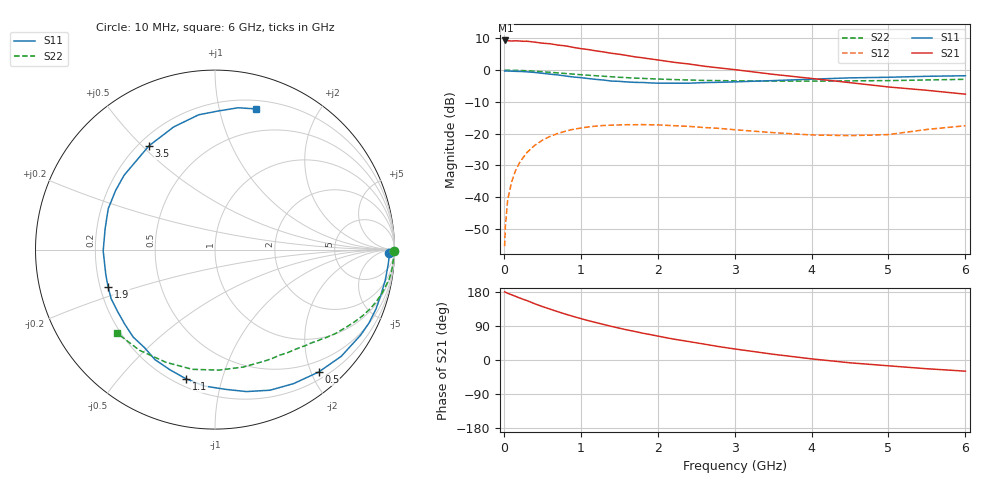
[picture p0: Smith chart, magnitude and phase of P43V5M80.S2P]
! SIEMENS Small Signal Semiconductors
! BFP182
! Si NPN RF Bipolar Junction Transistor in SOT143
! VCE = 3.5 V  IC = 0.8 mA
! Common Emitter S-Parameters:  March  1996
# GHz  S  MA  R  50
!  f  S11  S21  S12  S22
! GHz  MAG  ANG  MAG  ANG  MAG  ANG  MAG  ANG
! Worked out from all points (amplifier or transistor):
!   36 points, 10 MHz to 6 GHz, reference 50 ohm
!   highest |S21| = 9.3 dB at 20 MHz (marker M1)
!   |S21| within 3 dB of that: start of sweep to 1.13 GHz
!   unconditionally stable (mu >= 1): 2.769 GHz to end of sweep
!   at 250 MHz: K = 0.09, MSG = 18.3 dB, |S12| = -27.5 dB
!   at 1.4 GHz: K = 0.52, MSG = 11.3 dB, |S12| = -17.3 dB
!   at 6 GHz: K = 1.11, MAG = 2.9 dB, |S12| = -17.5 dB
!   S11 on the Smith chart (normalised r, x): 10 MHz: 49, -27; 500 MHz: 0.31, -2.12; 1.1 GHz: 0.24, -0.77; 1.9 GHz: 0.23, -0.16; 3.5 GHz: 0.24, +0.52; 6 GHz: 0.28, +1.30
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0.01  0.9692 -1.0  2.885 179.6  0.0017 85.5  0.9986 -0.3
0.02  0.9717 -2.0  2.934 179.1  0.0035 83.0  0.9999 -0.8
0.05  0.9682 -5.1  2.911 176.1  0.0091 89.3  0.9983 -1.8
0.1  0.964 -10.0  2.874 172.2  0.0172 83.3  0.9943 -3.7
0.15  0.9584 -15.5  2.897 168.2  0.0259 79.9  0.9931 -5.6
0.3  0.941 -30.4  2.852 156.8  0.0505 71.1  0.9777 -11.0
0.4  0.921 -40.2  2.762 148.5  0.0654 64.7  0.9626 -14.5
0.5  0.8937 -49.8  2.66 141.1  0.0788 58.5  0.9447 -17.8
0.6  0.8656 -59.6  2.604 134.3  0.0907 53.0  0.9263 -20.7
0.8  0.8102 -77.5  2.413 121.1  0.1094 43.1  0.8855 -26.1
1.1  0.7378 -102.6  2.107 103.7  0.128 30.4  0.8319 -32.8
1.3  0.6985 -118.6  1.931 93.6  0.1349 23.1  0.8018 -36.8
1.5  0.6672 -133.1  1.781 84.0  0.1374 17.1  0.7725 -40.4
1.9  0.6307 -160.9  1.505 67.2  0.1383 7.0  0.7338 -47.0
2.2  0.623 -179.4  1.335 55.4  0.1339 1.4  0.7113 -51.8
2.8  0.6441 149.4  1.085 35.2  0.1214 -6.1  0.6852 -62.2
3.5  0.6852 122.5  0.86 15.2  0.104 -7.4  0.6731 -76.5
4  0.7212 108.6  0.741 3.0  0.0956 -2.9  0.6717 -88.2
4.5  0.7566 96.9  0.636 -7.4  0.0933 3.0  0.6789 -100.7
5  0.7732 88.4  0.544 -15.3  0.0969 13.1  0.6848 -113.5
5.5  0.8007 80.7  0.482 -23.1  0.1167 16.0  0.7012 -126.9
6  0.8167 73.7  0.419 -29.5  0.1336 15.6  0.7178 -139.7
